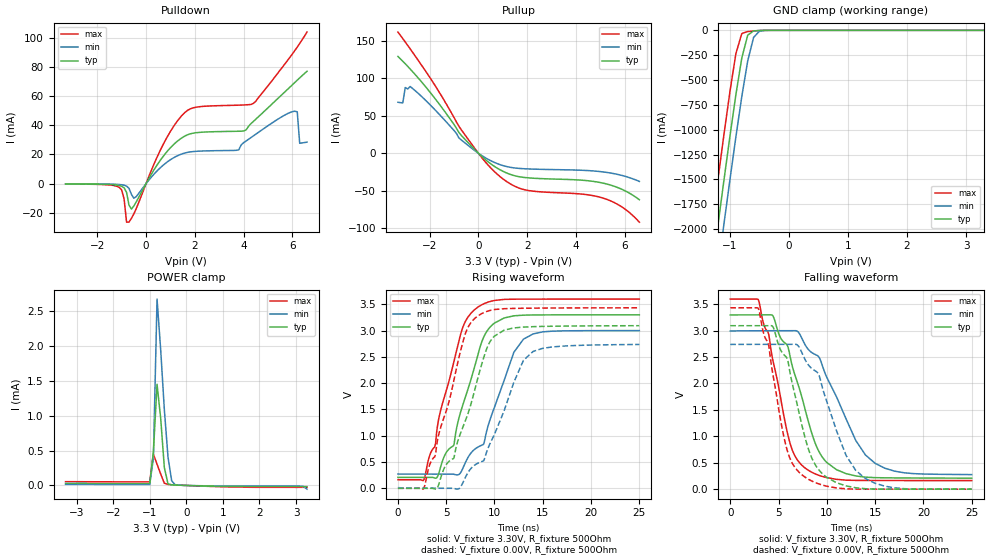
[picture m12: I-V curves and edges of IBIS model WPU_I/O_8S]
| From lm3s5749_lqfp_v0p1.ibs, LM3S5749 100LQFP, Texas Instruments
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[Model]   WPU_I/O_8S
Model_type   I/O
Vinl = 1.26
Vinh = 2.04
Vmeas = 1.65
| variable   typ   min   max
C_comp   9.739pF   9.739pF   9.803pF
[Model Spec]
Vinh+   1.91   1.78   2.04
Vinh-   1.90   1.76   2.03
Vinl+   1.40   1.27   1.54
Vinl-   1.39   1.26   1.53
| variable   typ   min   max
[Temperature Range]  25   85   -40
[Voltage Range]   3.3V   3.0V   3.6V
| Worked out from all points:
|   slope of the pulldown table from 0 to 0.495 V, typ, clamps not added: 35.8 ohm
|   slope of the pullup table from 0 to 0.495 V, typ, clamps not added: 35.8 ohm
|   GND clamp passes 1 mA (typ) near -0.48 V on its own axis
|   POWER clamp passes 1 mA (typ) near -0.71 V on its own axis
|   falling waveform, V_fixture 3.30V, R_fixture 500Ohm: 20-80 % time 2.89ns typ, 4.05ns min, 2.22ns max; typ from 3.3 V to 0.209 V
|   rising waveform, V_fixture 3.30V, R_fixture 500Ohm: 20-80 % time 2.69ns typ, 3.1ns min, 2.58ns max; typ from 0.208 V to 3.3 V
|   falling waveform, V_fixture 0.00V, R_fixture 500Ohm: 20-80 % time 2.49ns typ, 3.21ns min, 2.03ns max; typ from 3.09 V to 0 V
|   rising waveform, V_fixture 0.00V, R_fixture 500Ohm: 20-80 % time 3.02ns typ, 3.46ns min, 2.75ns max; typ from 0.001 V to 3.09 V
[Pulldown]
|  Voltage   I(typ)   I(min)   I(max)
-3.3V     -256.4uA   -145.5uA   -364.3uA
-1.1V     -1.272mA   -586.9uA   -2.565mA
-700mV    -14.71mA   -3.213mA   -26.31mA
-500mV    -15.24mA   -9.997mA   -20.64mA
600mV     16.38mA    11.14mA    23.43mA
1.5V      31.7mA     20.53mA    47.23mA
3.8V      35.88mA    23.14mA    53.74mA
4.4V      42.6mA     32.69mA    54.97mA
6.1V      69.26mA    49.6mA     91.12mA
6.2V      70.84mA    49.17mA    93.51mA
6.3V      72.42mA    27.66mA    95.98mA
6.6V      76.89mA    28.41mA    103.8mA
[Pullup]
|  Voltage   I(typ)   I(min)   I(max)
-3.3V     129.3mA    68.2mA     161.9mA
-3.1V     122.9mA    67.41mA    153.1mA
-3V       119.6mA    87.83mA    148.7mA
-2.8V     112.7mA    89.21mA    139.6mA
-1.8V     73.98mA    58.72mA    91.66mA
-700mV    23.82mA    17.72mA    31.27mA
300mV     -8.84mA    -6.3mA     -12.15mA
1V        -23.98mA   -16.37mA   -34.08mA
2V        -32.71mA   -20.86mA   -49.43mA
5.1V      -39.81mA   -24.88mA   -59.77mA
5.9V      -48.4mA    -29.75mA   -72.06mA
6.6V      -62.06mA   -37.61mA   -92.08mA
[GND Clamp]
|  Voltage   I(typ)   I(min)   I(max)
-3.3V     -11.73A    -12.14A    -11.32A
-1.4V     -2.85A     -3.29A     -2.391A
-1.3V     -2.393A    -2.835A    -1.933A
-1.2V     -1.942A    -2.383A    -1.481A
-1.1V     -1.496A    -1.937A    -1.038A
-1V       -1.061A    -1.498A    -612.1mA
-900mV    -646.5mA   -1.071A    -233.9mA
-800mV    -278.2mA   -665.9mA   -32.19mA
-700mV    -49.13mA   -307.7mA   -12.51mA
-600mV    -5.771mA   -70.87mA   -6.526mA
-500mV    -1.221mA   -8.174mA   -2.28mA
3.3V      2.312nA    7.026uA    -6.841uA
[POWER Clamp]
|  Voltage   I(typ)   I(min)   I(max)
-3.3V     29.71uA    15.87uA    54.94uA
-1V       27.67uA    14.78uA    51.22uA
-900mV    477.6uA    387.3uA    449.4uA
-800mV    1.453mA    2.675mA    305uA
-700mV    962.1uA    1.944mA    163.7uA
-600mV    254.6uA    1.086mA    31.4uA
-500mV    22.38uA    405.6uA    14.49uA
-400mV    7.783uA    67.02uA    10.49uA
-300mV    5.498uA    7.026uA    7.722uA
3.1V      -16.64uA   -9.952uA   -27.43uA
3.2V      -16.65uA   -12.25uA   -27.44uA
3.3V      -16.65uA   -53.27uA   -27.45uA
[Ramp]
| variable   typ   min   max
dV/dt_f   1.85/2.89n   1.63/4.05n   2.06/2.22n
dV/dt_r   1.85/3.02n   1.63/3.46n   2.06/2.75n
R_load = 500Ohm
[Falling Waveform]
V_fixture = 3.30V
V_fixture_min = 3.00V
V_fixture_max = 3.60V
R_fixture = 500Ohm
|   Time   V(typ)   V(min)   V(max)
0s        3.297V     2.993V     3.597V
2.9ns     3.298V     2.998V     3.588V
4.4ns     3.285V     2.998V     2.45V
6.2ns     2.507V     2.999V     863.5mV
7.8ns     1.474V     2.717V     393.5mV
8.9ns     822.8mV    2.539V     281.5mV
10ns      504.1mV    2.115V     218.2mV
13ns      250.1mV    920.3mV    165.8mV
15ns      218mV      489.3mV    164.4mV
25ns      208.5mV    275.7mV    162.4mV
[Rising Waveform]
V_fixture = 3.30V
V_fixture_min = 3.00V
V_fixture_max = 3.60V
R_fixture = 500Ohm
|   Time   V(typ)   V(min)   V(max)
0s        207.7mV    271.8mV    162.2mV
2.7ns     207.5mV    270.7mV    165.9mV
4.1ns     223mV      270.3mV    1.19V
5.8ns     823.8mV    267.1mV    2.412V
6.6ns     1.515V     332.8mV    2.996V
8.1ns     2.416V     762.7mV    3.421V
8.9ns     2.882V     848.2mV    3.509V
9.7ns     3.095V     1.392V     3.56V
13ns      3.293V     2.836V     3.597V
25ns      3.299V     2.999V     3.598V
[Falling Waveform]
V_fixture = 0.00V
V_fixture_min = 0.00V
V_fixture_max = 0.00V
R_fixture = 500Ohm
|   Time   V(typ)   V(min)   V(max)
0s        3.093V     2.739V     3.433V
2.9ns     3.093V     2.74V      3.423V
4ns       3.094V     2.74V      2.703V
4.4ns     3.079V     2.74V      2.187V
5.8ns     2.5V       2.741V     798.4mV
7.6ns     1.077V     2.508V     246.9mV
9.6ns     282mV      1.881V     74.67mV
12ns      61.67mV    635.6mV    6.05mV
14ns      8.398mV    200.8mV    317.7uV
25ns      42.17uV    193.1uV    23.99uV
[Rising Waveform]
V_fixture = 0.00V
V_fixture_min = 0.00V
V_fixture_max = 0.00V
R_fixture = 500Ohm
|   Time   V(typ)   V(min)   V(max)
0s        982.2uV    13.53mV    201.1uV
2.7ns     218.5uV    1.482mV    4.717mV
4ns       -9.375mV   1.191mV    805.7mV
5.8ns     575.1mV    -2.064mV   2.059V
7ns       1.294V     213.3mV    2.95V
8.2ns     2.045V     470mV      3.267V
10ns      2.895V     1.028V     3.399V
13ns      3.066V     2.434V     3.424V
14ns      3.074V     2.603V     3.426V
25ns      3.092V     2.735V     3.432V
